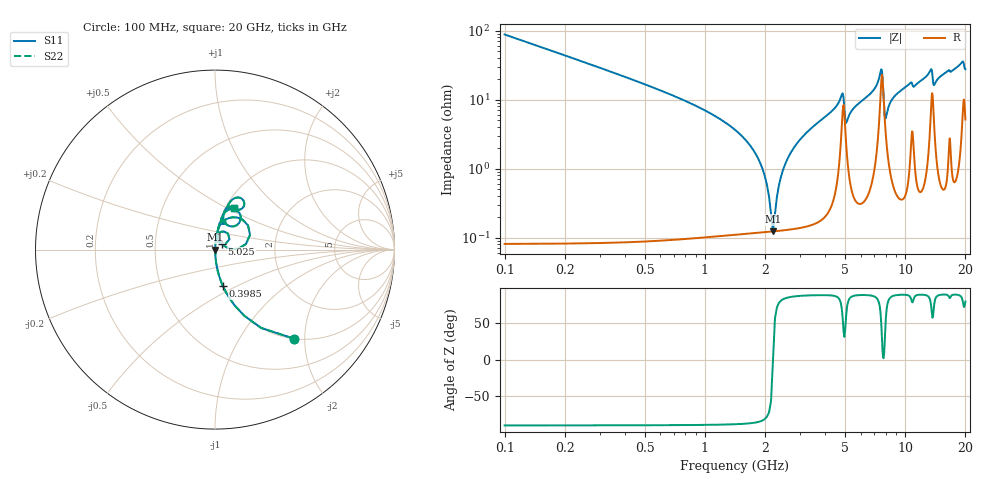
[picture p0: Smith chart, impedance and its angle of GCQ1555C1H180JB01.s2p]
!Murata Part Number: GCQ1555C1H180JB01
!These Parameters are Measured in Series Mode Connection
!Data Generated on Mar 13, 2026
!  o--ll--o
!Port1  Port2
!  o------o
!Operation Temp=25[degC], DC Bias Voltage=0[V]
!Freq. Start=100[MHz] Stop=20[GHz] 401[Steps]
# Hz S RI R 50
!Freq.(Hz) S11(Real) S11(Imag) S21(Real) S21(Imag) S12(Real) S12(Imag) S22(Real) S22(Imag)
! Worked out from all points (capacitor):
!   401 points, 100 MHz to 20 GHz, reference 50 ohm
!   read as one part in series: C = 18 pF near 199.5 MHz
!   lowest |Z| = 123 mohm at 2.189 GHz (marker M1)
!   series resonance near 2.189 GHz, so ESL is about 290 pH
!   S11 on the Smith chart (normalised r, x): 100 MHz: 1.00, -1.76; 398.5 MHz: 1.00, -0.43; 5.025 GHz: 1.07, +0.07; 20 GHz: 1.10, +0.54
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1e8  0.4378 -0.4957  0.5622 0.4957  0.5622 0.4957  0.4378 -0.4957
3.985e8  0.0447 -0.2048  0.9553 0.2048  0.9553 0.2048  0.0447 -0.2048
1.74175e9  0.00151 -0.0187  0.9985 0.0187  0.9985 0.0187  0.00151 -0.0187
1.94075e9  0.00129 -0.00983  0.9987 0.00983  0.9987 0.00983  0.00129 -0.00983
2.1895e9  0.00123 1.9e-06  0.9988 -1.9e-06  0.9988 -1.9e-06  0.00123 1.9e-06
2.43825e9  0.00135 0.00884  0.9987 -0.00884  0.9987 -0.00884  0.00135 0.00884
2.63725e9  0.00154 0.0154  0.9985 -0.0154  0.9985 -0.0154  0.00154 0.0154
3.43325e9  0.00308 0.0393  0.9969 -0.0393  0.9969 -0.0393  0.00308 0.0393
4.82625e9  0.0497 0.1012  0.9503 -0.1012  0.9503 -0.1012  0.0497 0.1012
5.02525e9  0.037 0.0315  0.963 -0.0315  0.963 -0.0315  0.037 0.0315
5.12475e9  0.0175 0.0447  0.9825 -0.0447  0.9825 -0.0447  0.0175 0.0447
6.7665e9  0.0208 0.1221  0.9792 -0.1221  0.9792 -0.1221  0.0208 0.1221
7.61225e9  0.1843 0.1346  0.8157 -0.1346  0.8157 -0.1346  0.1843 0.1346
7.91075e9  0.0507 0.0214  0.9493 -0.0214  0.9493 -0.0214  0.0507 0.0214
8.01025e9  0.0318 0.0419  0.9682 -0.0419  0.9682 -0.0419  0.0318 0.0419
8.657e9  0.0164 0.101  0.9836 -0.101  0.9836 -0.101  0.0164 0.101
1.005e10  0.0264 0.1472  0.9736 -0.1472  0.9736 -0.1472  0.0264 0.1472
1.338325e10  0.1034 0.2251  0.8966 -0.2251  0.8966 -0.2251  0.1034 0.2251
1.39305e10  0.067 0.138  0.933 -0.138  0.933 -0.138  0.067 0.138
1.67165e10  0.0847 0.2304  0.9153 -0.2304  0.9153 -0.2304  0.0847 0.2304
1.93035e10  0.1422 0.2873  0.8578 -0.2873  0.8578 -0.2873  0.1422 0.2873
2e10  0.1084 0.2299  0.8916 -0.2299  0.8916 -0.2299  0.1084 0.2299
